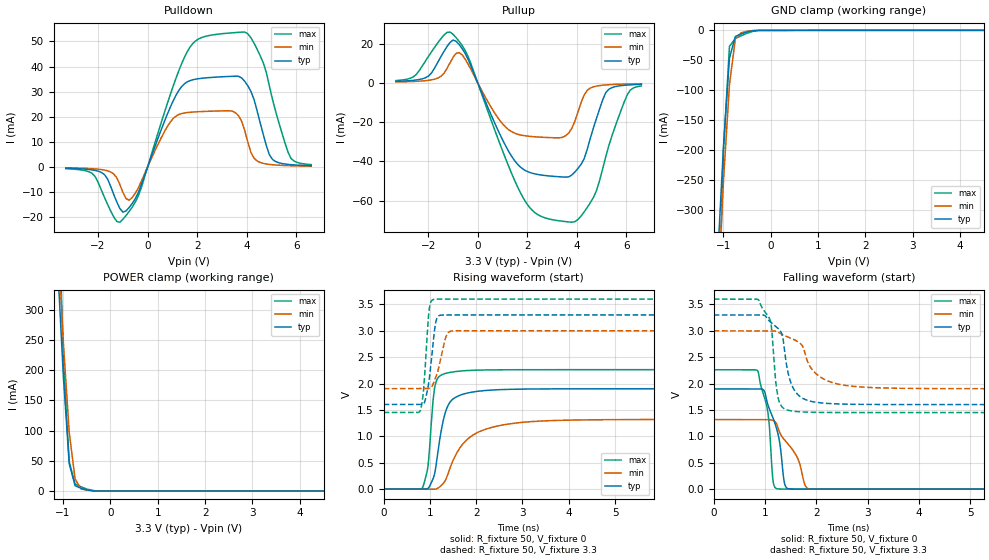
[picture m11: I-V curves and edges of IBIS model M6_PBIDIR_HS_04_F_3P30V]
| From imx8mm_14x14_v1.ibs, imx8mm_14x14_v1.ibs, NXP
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[Model] M6_PBIDIR_HS_04_F_3P30V
Model_type I/O
Vinl  =  0.99
Vinh  =  2.31
Vmeas =  1.65
| Capacitance   typ   min   max
C_comp   1.08818991111e-12   1.03117834871e-12   1.10439570077e-12
| Variables   typ   min   max
[GND Clamp Reference]   0   0   0
[POWER Clamp Reference]   3.3   3   3.6
[Pulldown Reference]   0   0   0
[Pullup Reference]   3.3   3   3.6
[Temperature Range]   25   125   -40
[Voltage Range]   3.3   3   3.6
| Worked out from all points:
|   slope of the pulldown table from 0 to 0.495 V, typ, clamps not added: 36.9 ohm
|   slope of the pullup table from 0 to 0.495 V, typ, clamps not added: 33.1 ohm
|   GND clamp passes 1 mA (typ) near -0.39 V on its own axis
|   POWER clamp passes 1 mA (typ) near -0.44 V on its own axis
|   falling waveform, R_fixture 50, V_fixture 0: 20-80 % time 258ps typ, 434ps min, 165ps max; typ from 1.9 V to 0.002 V
|   falling waveform, R_fixture 50, V_fixture 3.3: 20-80 % time 216ps typ, 419ps min, 120ps max; typ from 3.3 V to 1.6 V
|   rising waveform, R_fixture 50, V_fixture 0: 20-80 % time 239ps typ, 614ps min, 123ps max; typ from 0.002 V to 1.9 V
|   rising waveform, R_fixture 50, V_fixture 3.3: 20-80 % time 132ps typ, 181ps min, 97ps max; typ from 1.6 V to 3.3 V
[GND Clamp]
| Voltage   I(typ)   I(min)   I(max)
-3.3V     -7.236A    -6.565A    -8.004A
-1.117V   -380.4mA   -438.7mA   -546.7mA
-993.1mV  -191mA     -249.4mA   -198.9mA
-869mV    -46.61mA   -90.79mA   -26.93mA
-744.8mV  -10.31mA   -14.37mA   -13.71mA
-620.7mV  -5.945mA   -4.193mA   -9.059mA
-372.4mV  -659.7uA   -360.2uA   -1.673mA
-248.3mV  -143.8uA   -94.2uA    -265.5uA
6.6V      0A         0A         0A
[POWER Clamp]
| Voltage   I(typ)   I(min)   I(max)
-3.3V     7.237A     6.564A     8.009A
-1.117V   380.7mA    433.6mA    553.5mA
-993.1mV  190.7mA    247mA      219.9mA
-869mV    45.33mA    97.36mA    48.38mA
-744.8mV  8.677mA    19.82mA    11.82mA
-620.7mV  4.425mA    3.499mA    6.828mA
-372.4mV  215.5uA    293.3uA    764.6uA
-248.3mV  4.273uA    22.4uA     51.08uA
6.6V      0A         0A         0A
[Pulldown]
| Voltage   I(typ)   I(min)   I(max)
-3.3V     -504.5uA   -348.9uA   -699.6uA
-2.234V   -1.177mA   -696.7uA   -2.583mA
-1.738V   -3.068mA   -1.25mA    -12.18mA
-1.117V   -16.59mA   -7.062mA   -22.02mA
-620.7mV  -14.56mA   -12.2mA    -15.99mA
910.3mV   23.7mA     17.82mA    28.7mA
1.707V    34.39mA    21.79mA    47.68mA
3.797V    35.45mA    18.16mA    53.73mA
4.293V    26.89mA    3.485mA    49.33mA
5.038V    3.002mA    871.4uA    26.92mA
5.783V    903.1uA    485.4uA    3.433mA
6.6V      512.6uA    324.7uA    916.9uA
[Pullup]
| Voltage   I(typ)   I(min)   I(max)
-3.3V     775.3uA    487.4uA    1.181mA
-2.607V   1.309mA    735uA      3.011mA
-1.986V   3.506mA    1.318mA    13.54mA
-993.1mV  21.85mA    13.1mA     24.75mA
-620.7mV  17.35mA    14.17mA    18.9mA
1.024V    -29.57mA   -21.17mA   -35.34mA
1.934V    -44.73mA   -26.99mA   -60.67mA
3.797V    -46.9mA    -23.15mA   -70.97mA
4.417V    -33.81mA   -3.799mA   -63.46mA
5.162V    -5.034mA   -1.021mA   -37.7mA
6.031V    -1.089mA   -543.8uA   -6.056mA
6.6V      -731.8uA   -415.3uA   -1.532mA
[Ramp]
dV/dt_r   1.13914/0.239221n  0.791175/0.614129n  1.35569/0.122717n
dV/dt_f   1.01801/0.21596n  0.657879/0.419368n  1.28879/0.120301n
R_load = 50
[Falling Waveform]
R_fixture = 50
V_fixture = 0
V_fixture_min = 0
V_fixture_max = 0
| Time   V(typ)   V(min)   V(max)
0s        1.901V     1.32V      2.262V
856.7ps   1.901V     1.32V      2.239V
1.058ns   1.591V     1.32V      1.434V
1.165ns   1.326V     1.302V     108.4mV
1.276ns   932.5mV    1.093V     4.98mV
1.35ns    304.1mV    969.1mV    3.548mV
1.428ns   19.54mV    879mV      3.414mV
1.794ns   2.433mV    49.39mV    3.129mV
1.993ns   2.306mV    2.004mV    3.129mV
333.3ns   2.091mV    1.408mV    2.913mV
[Falling Waveform]
R_fixture = 50
V_fixture = 3.3
V_fixture_min = 3
V_fixture_max = 3.6
| Time   V(typ)   V(min)   V(max)
0s        3.3V       3V         3.6V
873.8ps   3.3V       3V         3.585V
1.112ns   3.16V      3.001V     3.151V
1.21ns    3.083V     2.991V     2.016V
1.302ns   2.991V     2.945V     1.601V
1.454ns   2.181V     2.88V      1.495V
1.575ns   1.871V     2.829V     1.475V
2.191ns   1.627V     2.064V     1.454V
5.667ns   1.603V     1.904V     1.452V
333.3ns   1.603V     1.904V     1.452V
[Rising Waveform]
R_fixture = 50
V_fixture = 0
V_fixture_min = 0
V_fixture_max = 0
| Time   V(typ)   V(min)   V(max)
0s        2.091mV    1.408mV    2.913mV
840.3ps   1.503mV    1.381mV    27.38mV
959.2ps   14.63mV    1.171mV    444.9mV
1.072ns   205.4mV    -458.2uV   1.716V
1.189ns   809.9mV    27.35mV    2.124V
1.319ns   1.411V     144.8mV    2.187V
1.475ns   1.688V     492mV      2.217V
1.845ns   1.827V     970.5mV    2.248V
2.453ns   1.882V     1.194V     2.26V
333.3ns   1.901V     1.32V      2.262V
[Rising Waveform]
R_fixture = 50
V_fixture = 3.3
V_fixture_min = 3
V_fixture_max = 3.6
| Time   V(typ)   V(min)   V(max)
0s        1.603V     1.904V     1.452V
787.5ps   1.603V     1.904V     1.479V
860.2ps   1.616V     1.904V     1.86V
959.5ps   1.936V     1.904V     3.173V
992.8ps   2.14V      1.909V     3.455V
1.116ns   3.116V     2.094V     3.597V
1.208ns   3.289V     2.365V     3.599V
1.376ns   3.299V     2.944V     3.599V
1.667ns   3.299V     2.999V     3.599V
333.3ns   3.3V       3V         3.6V
